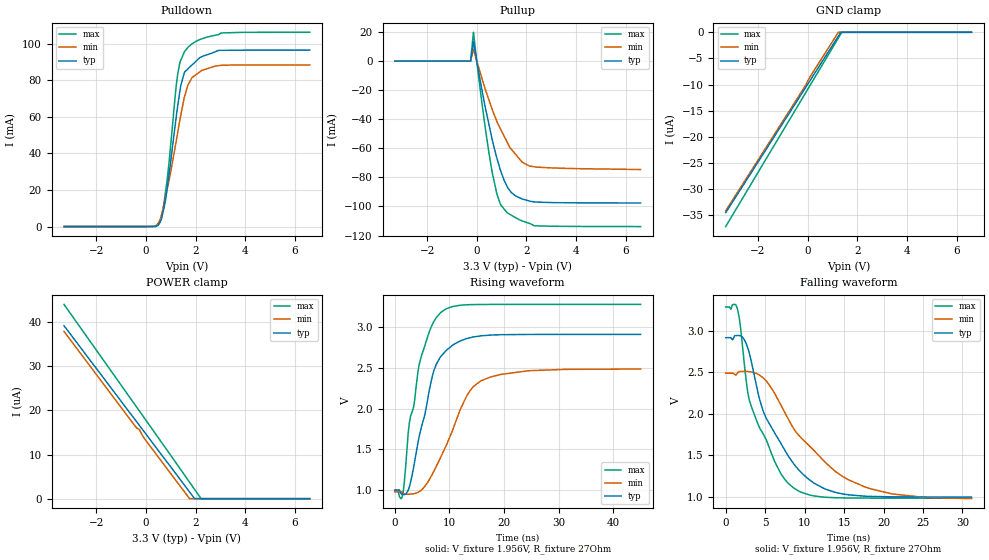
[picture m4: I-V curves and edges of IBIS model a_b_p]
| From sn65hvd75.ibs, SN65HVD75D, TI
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|   a_b Model
[Model]   a_b_p
Model_type   I/O
Polarity   Non-Inverting
Enable   Active-High
Vinl = 0.8
Vinh = 2.0
Vmeas = 1.65
Vref = 1.65
Cref = 50pF
Rref = 27
|   typ   min   max
|   (nom PVT)   (fast PVT)   (slow PVT)
C_comp   1.371e-11   1.433e-11   1.572e-11
|ON state : BUFFER OUTPUT TURNED HIGH
|C_comp   1.371e-11   1.433e-11   1.572e-11
|OFF state: BUFFER IN HIGH IMPEDANCE
|C_comp   1.142e-11   1.069e-11   1.206e-11
| Where nom  PVT is Nominal Process, 3.3V, 27C
|   Fast PVT is Strong Process,  3.6V, -40C
|   Slow PVT is Weak Process,   3V, 125C
[Voltage Range]   3.3   3   3.6
|Ambient Temperature   25   125   -40
|Junction Temperature
[Temperature Range]   27   125   -40
[Pullup Reference]   3.3   3   3.6
[Pulldown Reference]   0   0   0
[Power Clamp Reference]   3.3   3   3.6
[GND Clamp Reference]   0   0   0
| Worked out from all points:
|   slope of the pulldown table from 0 to 0.495 V, typ, clamps not added: 482 ohm
|   slope of the pullup table from 0 to 0.495 V, typ, clamps not added: 11.3 ohm
|   falling waveform, V_fixture 1.956V, R_fixture 27Ohm: 20-80 % time 5.29ns typ, 7.74ns min, 4.01ns max; typ from 2.92 V to 0.998 V
|   rising waveform, V_fixture 1.956V, R_fixture 27Ohm: 20-80 % time 3.79ns typ, 5.93ns min, 3.55ns max; typ from 0.997 V to 2.91 V
[Pulldown]
|   Voltage   I(typ)   I(min)   I(max)
-3.3V     0A         0A         0A
478.8mV   881.8uA    1.608mA    490.4uA
633.6mV   4.473mA    6.787mA    5.518mA
849.6mV   20.36mA    20.02mA    24.85mA
1.202V    57.94mA    45.29mA    74.75mA
1.285V    66.34mA    51.87mA    83.81mA
1.399V    76.97mA    60.61mA    90.81mA
1.554V    84.49mA    70.97mA    95.7mA
1.854V    88.36mA    81.44mA    99.95mA
2.168V    92.42mA    84.62mA    102.3mA
2.934V    96.41mA    88.05mA    105.1mA
6.6V      96.53mA    88.41mA    106.3mA
[GND Clamp]
|   Voltage   I(typ)   I(min)   I(max)
-3.3V     -34.52uA   -34.17uA   -37.17uA
-162mV    -11.18uA   -10.75uA   -12.24uA
111mV     -9.145uA   -8.427uA   -10.07uA
1.239V    -749.7nA   -4.43nA    -1.103uA
1.337V    -22.88nA   0A         -325.6nA
1.375V    0A         0A         -17.18nA
6.6V      0A         0A         0A
[Pullup]
|   Voltage   I(typ)   I(min)   I(max)
-3.3V     0A         0A         0A
-248.4mV  0A         0A         0A
-133.2mV  13.34mA    8.273mA    19.82mA
64.8mV    -6.244mA   -3.735mA   -9.275mA
342mV     -31.73mA   -19.41mA   -45.91mA
633.6mV   -54.97mA   -33.82mA   -77.49mA
802.8mV   -66.31mA   -41.19mA   -90.85mA
939.6mV   -74.34mA   -46.13mA   -97.84mA
1.213V    -85.9mA    -55.41mA   -104.1mA
1.554V    -92.65mA   -63.94mA   -107.6mA
2.115V    -96.23mA   -72.14mA   -111.7mA
6.6V      -97.64mA   -74.6mA    -113.8mA
[POWER Clamp]
|   Voltage   I(typ)   I(min)   I(max)
-3.3V     39.17uA    37.88uA    43.99uA
-378mV    17.44uA    16.03uA    20.77uA
-264mV    16.59uA    15.67uA    19.86uA
-150mV    15.75uA    14.42uA    18.96uA
6mV       14.58uA    13.11uA    17.71uA
1.758V    1.511uA    17.98nA    3.717uA
1.96V     1.728nA    0A         2.097uA
2.221V    0A         0A         11.53nA
6.6V      0A         0A         0A
[Ramp]
R_load = 27
|   typ   min   max
dV/dt_r   1.32253/4.34455e-09   0.977857/7.14186e-09   1.5873/3.91311e-09
dV/dt_f   1.15015/5.29663e-09   0.908153/7.77085e-09   1.38004/4.01336e-09
[Falling Waveform]
V_fixture = 1.956V
V_fixture_min = 1.731V
V_fixture_max = 2.134V
R_fixture = 27Ohm
C_fixture = 0F
|   Time   V(typ)   V(min)   V(max)
0s        2.915V     2.488V     3.285V
1.5ns     2.941V     2.49V      3.258V
2.44ns    2.878V     2.51V      2.53V
3ns       2.728V     2.506V     2.165V
4.79ns    2.022V     2.428V     1.752V
6.94ns    1.653V     2.115V     1.289V
8.58ns    1.403V     1.826V     1.11V
12.4ns    1.104V     1.437V     997.8mV
17.62ns   1.009V     1.121V     986mV
31.14ns   998.1mV    978.9mV    984.8mV
[Rising Waveform]
V_fixture = 1.956V
V_fixture_min = 1.731V
V_fixture_max = 2.134V
R_fixture = 27Ohm
C_fixture = 0F
|   Time   V(typ)   V(min)   V(max)
0s        996.9mV    973.6mV    983.5mV
1.44ns    940.4mV    962.3mV    940mV
2.63ns    1.028V     944.5mV    1.807V
3.47ns    1.288V     950.8mV    2.03V
4.9ns     1.782V     996.3mV    2.654V
7.08ns    2.453V     1.219V     3.065V
8.62ns    2.657V     1.432V     3.195V
13.13ns   2.862V     2.151V     3.279V
15.82ns   2.897V     2.344V     3.283V
45ns      2.914V     2.487V     3.284V
